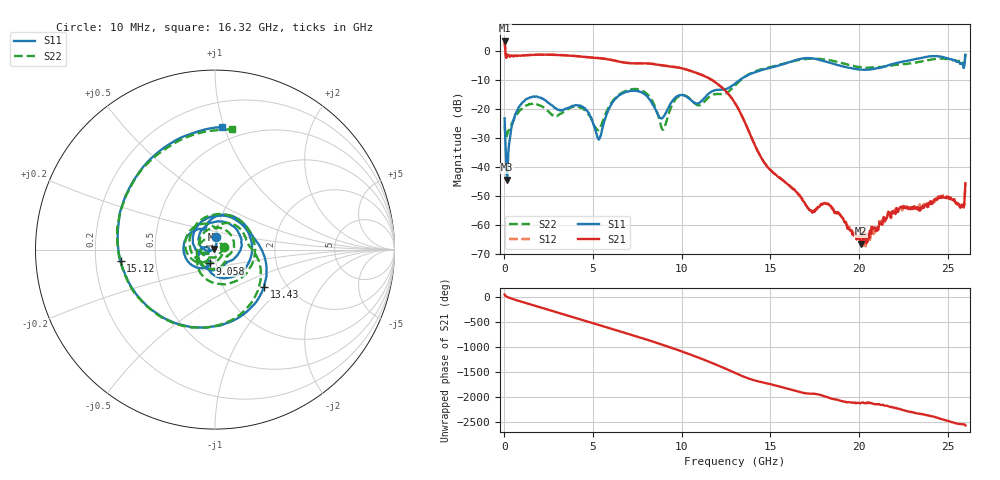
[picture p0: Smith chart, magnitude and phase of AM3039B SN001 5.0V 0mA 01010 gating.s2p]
!Agilent Technologies,E8364B,MY43040894,A.07.50.67
!Agilent E8364B: A.07.50.67
!Date: Tuesday, June 28, 2016 08:05:39
!Correction: S11(Full 2 Port(1,2))
!S21(Full 2 Port(1,2))
!S12(Full 2 Port(1,2))
!S22(Full 2 Port(1,2))
!S2P File: Measurements: S11, S21, S12, S22:
# Hz S  dB  R 50
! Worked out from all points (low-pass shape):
!   1601 points, 10 MHz to 26 GHz, reference 50 ohm
!   highest |S21| = 3.63 dB at 10 MHz (marker M1); lowest = -66.3 dB at 20.09 GHz (marker M2)
!   |S21| within 3 dB of the highest: start of sweep to 44.37 MHz
!   lowest |S11| = -44.3 dB at 156.2 MHz (marker M3), VSWR 1.01, Z = 49.5 + j0.336 ohm
!   |S11| at or under -10 dB: start of sweep to 13.26 GHz
!   |S22| runs from -29.8 to -0.8 dB; largest |S21 - S12| = 0.026
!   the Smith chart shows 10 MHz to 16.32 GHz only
!   S11 on the Smith chart (normalised r, x): 10 MHz: 1.00, +0.14; 9.058 GHz: 0.94, -0.15; 13.43 GHz: 1.54, -0.73; 15.12 GHz: 0.31, -0.06; 16.32 GHz: 0.38, +0.98
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1e7  -23.19 85.6  3.63 40.6  3.70 41.5  -25.68 17.9
1.561938e8  -44.26 146.4  -1.40 -5.3  -1.33 -5.1  -28.72 -62.4
8.54675e8  -18.91 142.7  -1.52 -90.7  -1.47 -90.6  -20.43 161.5
1.634375e9  -15.61 63.0  -1.27 -172.9  -1.23 -172.7  -17.94 68.0
2.657731e9  -18.58 -25.1  -1.24 80.4  -1.17 80.6  -21.77 -22.4
3.469919e9  -19.79 -62.5  -1.45 -4.7  -1.41 -4.7  -20.36 -64.3
4.347081e9  -19.04 -135.9  -1.88 -97.8  -1.85 -97.7  -19.56 -162.0
5.809019e9  -21.05 -169.0  -2.77 104.4  -2.73 104.6  -20.22 -133.0
7.563344e9  -13.85 -16.0  -4.20 -82.2  -4.16 -82.2  -13.18 -30.7
8.684162e9  -22.18 -119.9  -4.69 148.9  -4.64 148.8  -22.37 -162.6
9.057769e9  -21.77 -108.8  -5.05 105.3  -5.01 105.2  -25.77 -129.2
1.3005e10  -11.17 -7.3  -17.88 -77.8  -17.88 -78.5  -11.81 -16.1
1.342734e10  -9.29 -37.4  -22.71 -142.4  -22.72 -143.2  -9.47 -46.3
1.511669e10  -5.52 -173.0  -41.64 48.2  -41.59 48.4  -5.30 177.5
1.631872e10  -3.30 86.8  -47.70 -63.1  -47.48 -63.8  -3.40 82.0
1.734208e10  -2.46 -12.3  -55.50 -134.7  -55.32 -132.0  -2.58 -6.7
1.836544e10  -4.01 -106.5  -53.20 142.4  -53.22 141.1  -3.14 -95.4
2.008728e10  -6.32 122.6  -66.32 43.5  -64.63 37.8  -5.49 132.7
2.167916e10  -4.79 15.9  -55.66 -23.2  -56.05 -29.1  -5.07 22.1
2.312486e10  -2.81 -92.5  -53.73 -152.5  -54.29 -151.5  -3.99 -82.5
2.422943e10  -1.70 177.8  -51.20 131.8  -52.12 130.0  -2.74 -166.6
2.6e10  -1.40 -21.7  -45.52 -42.3  -45.67 -38.1  -0.85 8.0
